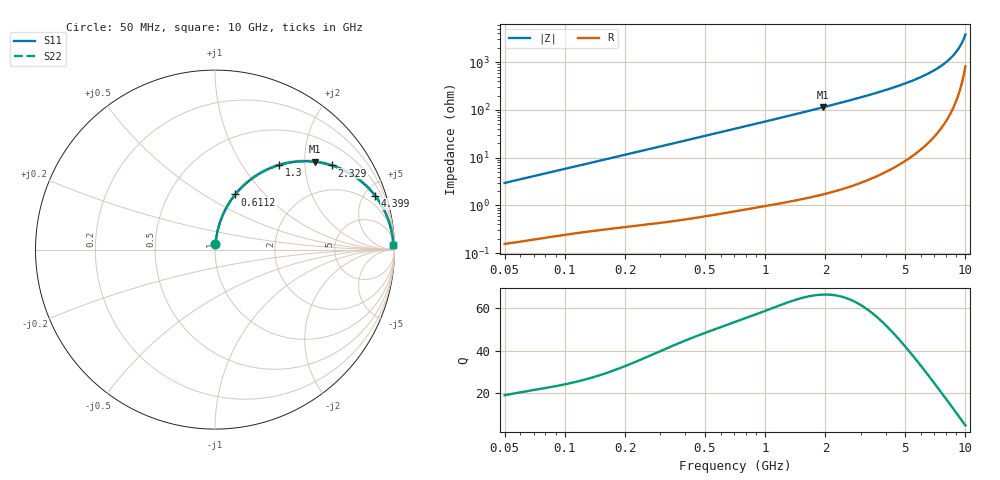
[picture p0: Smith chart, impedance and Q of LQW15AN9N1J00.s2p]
!Murata Part Number: LQW15AN9N1J00
!These Parameters are Measured in Series Mode Connection
!  o--[Z]--o
!Port1  Port2
!  o-------o
!Freq. Start=50[MHz] Stop=10[GHz], 401[Steps]
# Hz S RI R 50
!Freq.(Hz)	S 11(Real)	S 11(Imag)	S 21(Real)	S 21(Imag)	S 12(Real)	S 12(Imag)	S 22(Real)	S 22(Imag)
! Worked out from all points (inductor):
!   401 points, 50 MHz to 10 GHz, reference 50 ohm
!   read as one part in series: L = 9.38 nH near 51.34 MHz
!   highest Q = 66.6 at 1.935 GHz (marker M1), where L = 9.27 nH
!   S11 on the Smith chart (normalised r, x): 50 MHz: 1.00, +0.06; 611.2 MHz: 1.01, +0.70; 1.3 GHz: 1.02, +1.49; 2.329 GHz: 1.04, +2.75; 4.399 GHz: 1.12, +5.93; 10 GHz: 17, +74
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5e7  0.00243 0.0295  0.9976 -0.0295  0.9976 -0.0295  0.00243 0.0295
1.214486e8  0.00763 0.0698  0.9924 -0.0698  0.9924 -0.0698  0.00763 0.0698
2.949953e8  0.0317 0.163  0.9683 -0.163  0.9683 -0.163  0.0317 0.163
4.38927e8  0.0636 0.2335  0.9364 -0.2335  0.9364 -0.2335  0.0636 0.2335
6.112328e8  0.1131 0.3071  0.8869 -0.3071  0.8869 -0.3071  0.1131 0.3071
7.071068e8  0.1444 0.3423  0.8556 -0.3423  0.8556 -0.3423  0.1444 0.3423
9.589462e8  0.2343 0.4151  0.7657 -0.4151  0.7657 -0.4151  0.2343 0.4151
1.300479e9  0.3593 0.4719  0.6407 -0.4719  0.6407 -0.4719  0.3593 0.4719
1.717543e9  0.4969 0.4925  0.5031 -0.4925  0.5031 -0.4925  0.4969 0.4925
1.934999e9  0.5585 0.4891  0.4415 -0.4891  0.4415 -0.4891  0.5585 0.4891
2.329253e9  0.6521 0.4688  0.3479 -0.4688  0.3479 -0.4688  0.6521 0.4688
3.158828e9  0.7868 0.4013  0.2132 -0.4013  0.2132 -0.4013  0.7868 0.4013
4.171863e9  0.8789 0.3164  0.1211 -0.3164  0.1211 -0.3164  0.8789 0.3164
4.398862e9  0.8929 0.299  0.1071 -0.299  0.1071 -0.299  0.8929 0.299
5.225452e9  0.931 0.2412  0.069 -0.2412  0.069 -0.2412  0.931 0.2412
6.045081e9  0.9552 0.1919  0.0448 -0.1919  0.0448 -0.1919  0.9552 0.1919
6.810442e9  0.9702 0.1519  0.0298 -0.1519  0.0298 -0.1519  0.9702 0.1519
7.571744e9  0.9802 0.1166  0.0198 -0.1166  0.0198 -0.1166  0.9802 0.1166
8.307378e9  0.9867 0.0861  0.0133 -0.0861  0.0133 -0.0861  0.9867 0.0861
8.876195e9  0.9901 0.0643  0.00991 -0.0643  0.00991 -0.0643  0.9901 0.0643
9.359165e9  0.9921 0.047  0.00792 -0.047  0.00792 -0.047  0.9921 0.047
1e10  0.9937 0.0255  0.0063 -0.0255  0.0063 -0.0255  0.9937 0.0255
